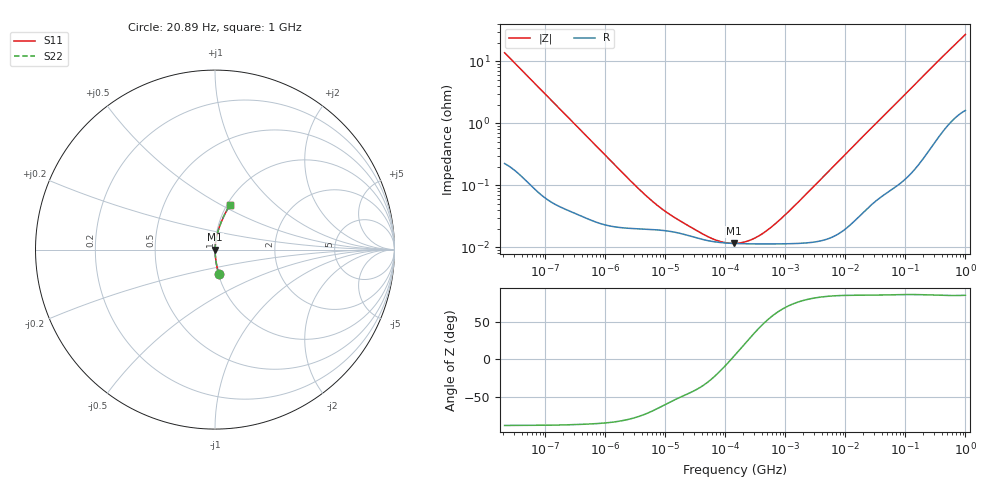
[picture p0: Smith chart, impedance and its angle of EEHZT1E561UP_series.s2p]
!  *** S-Parameter ***
!  Copyright (C) Panasonic Industry Co., Ltd.
!  Conductive Polymer Hybrid Aluminum Electrolytic Capacitor
!  Parts No. EEHZT1E561UP
!  Connection Mode : Series
!  1  o---||---o  2
!  GND o--------o GND
!  Conditions : Temperature = 20   DC Bias = 0 V
! Frequency Range : 20.9Hz  -  1GHz  [ 385 Steps ]
# Hz S RI R 50
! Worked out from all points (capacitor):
!   385 points, 20.89 Hz to 1 GHz, reference 50 ohm
!   read as one part in series: C = 549 uF near 21.88 Hz
!   lowest |Z| = 11.5 mohm at 138 kHz (marker M1)
!   series resonance near 124.4 kHz, so ESL is about 3 nH
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20.89296  0.0209 -0.1352  0.9791 0.1352  0.9791 0.1352  0.0209 -0.1352
34.67369  0.00855 -0.0831  0.9915 0.0831  0.9915 0.0831  0.00855 -0.0831
66.06934  0.00283 -0.0443  0.9972 0.0443  0.9972 0.0443  0.00283 -0.0443
398.1072  0.000374 -0.0075  0.9996 0.0075  0.9996 0.0075  0.000374 -0.0075
3019.952  0.000201 -0.00101  0.9998 0.00101  0.9998 0.00101  0.000201 -0.00101
7585.776  0.00019 -0.000421  0.9998 0.000421  0.9998 0.000421  0.00019 -0.000421
14454.4  0.000175 -0.000242  0.9998 0.000242  0.9998 0.000242  0.000175 -0.000242
50118.72  0.000128 -7.71e-05  0.9999 7.71e-05  0.9999 7.71e-05  0.000128 -7.71e-05
83176.38  0.000119 -3.2e-05  0.9999 3.2e-05  0.9999 3.2e-05  0.000119 -3.2e-05
138038.4  0.000115 8.26e-06  0.9999 -8.26e-06  0.9999 -8.26e-06  0.000115 8.26e-06
144544  0.000115 1.19e-05  0.9999 -1.19e-05  0.9999 -1.19e-05  0.000115 1.19e-05
190546.1  0.000114 3.49e-05  0.9999 -3.49e-05  0.9999 -3.49e-05  0.000114 3.49e-05
251188.6  0.000113 6.07e-05  0.9999 -6.07e-05  0.9999 -6.07e-05  0.000113 6.07e-05
331131.1  0.000113 9.12e-05  0.9999 -9.12e-05  0.9999 -9.12e-05  0.000113 9.12e-05
457088.2  0.000113 0.000136  0.9999 -0.000136  0.9999 -0.000136  0.000113 0.000136
912010.8  0.000114 0.000288  0.9999 -0.000288  0.9999 -0.000288  0.000114 0.000288
2754229  0.000121 0.000883  0.9999 -0.000883  0.9999 -0.000883  0.000121 0.000883
5.248075e7  0.00104 0.0158  0.999 -0.0158  0.999 -0.0158  0.00104 0.0158
1.380384e8  0.0034 0.0407  0.9966 -0.0407  0.9966 -0.0407  0.0034 0.0407
2.884032e8  0.0114 0.0827  0.9886 -0.0827  0.9886 -0.0827  0.0114 0.0827
5.495409e8  0.0328 0.1486  0.9672 -0.1486  0.9672 -0.1486  0.0328 0.1486
1e9  0.082 0.2463  0.918 -0.2463  0.918 -0.2463  0.082 0.2463
